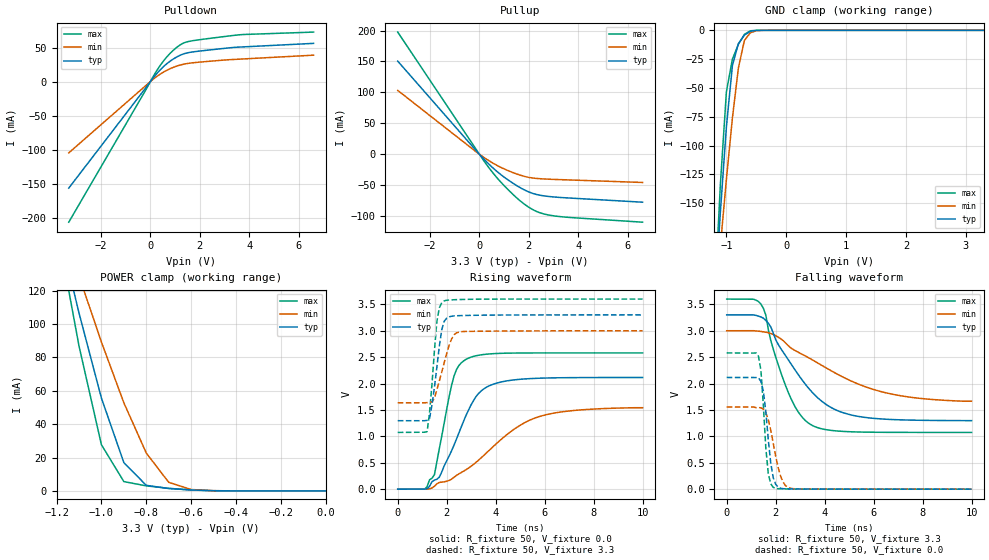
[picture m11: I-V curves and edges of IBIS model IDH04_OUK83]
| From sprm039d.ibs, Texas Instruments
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[Model]   IDH04_OUK83
Model_type   I/O
Vinh = 2.00
Vinl = 0.80
Enable   Active-Low
Polarity   Non-Inverting
| signals   A, GZ, Y
Vmeas = 1.5
|   typ   min   max
C_comp   2.356p   2.266p   2.394p
|   typ   min   max
[Temperature Range]   25   -40   125
|   typ   min   max
[Voltage Range]   3.30V   3.00V   3.60V
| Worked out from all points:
|   slope of the pulldown table from 0 to 0.495 V, typ, clamps not added: 23.8 ohm
|   slope of the pullup table from 0 to 0.495 V, typ, clamps not added: 24.4 ohm
|   GND clamp passes 1 mA (typ) near -0.61 V on its own axis
|   POWER clamp passes 1 mA (typ) near -0.65 V on its own axis
|   rising waveform, R_fixture 50, V_fixture 0.0: 20-80 % time 1.24ns typ, 2.52ns min, 658ps max; typ from 0 V to 2.12 V
|   falling waveform, R_fixture 50, V_fixture 3.3: 20-80 % time 1.85ns typ, 3.23ns min, 1.1ns max; typ from 3.3 V to 1.3 V
|   rising waveform, R_fixture 50, V_fixture 3.3: 20-80 % time 331ps typ, 486ps min, 260ps max; typ from 1.3 V to 3.3 V
|   falling waveform, R_fixture 50, V_fixture 0.0: 20-80 % time 285ps typ, 427ps min, 226ps max; typ from 2.12 V to 0 V
[Pulldown]
|   Voltage   I(typ)   I(min)   I(max)
-3.3V     -156.5mA   -104.8mA   -206.6mA
-200mV    -9.762mA   -6.342mA   -13.16mA
200mV     9.308mA    5.91mA     12.77mA
600mV     24.27mA    15.38mA    33.46mA
800mV     30.04mA    19mA       41.54mA
1.1V      36.8mA     23.15mA    51.22mA
1.3V      40.12mA    25.17mA    55.93mA
1.6V      42.95mA    27.12mA    59.33mA
3.5V      50.51mA    32.76mA    68.38mA
6.6V      56.15mA    38.81mA    72.73mA
[GND_clamp]
|   Voltage   I(typ)   I(min)   I(max)
-3.3V     -2.124A    -1.605A    -2.753A
-1.2V     -237.7mA   -246.3mA   -236.7mA
-1.1V     -157mA     -186.6mA   -132.9mA
-1V       -83.63mA   -129.2mA   -53.23mA
-900mV    -30.57mA   -76.17mA   -24.99mA
-800mV    -11.54mA   -32.67mA   -12.1mA
-700mV    -4.229mA   -8.865mA   -3.556mA
-600mV    -824.6uA   -2.094mA   -405.8uA
-500mV    -75.44uA   -369.7uA   -18.94uA
-400mV    -4.212uA   -45.39uA   -421.8nA
3.3V      310.9pA    1.955uA    0A
[Pullup]
|   Voltage   I(typ)   I(min)   I(max)
-3.3V     150.6mA    103.2mA    197.6mA
-200mV    9.015mA    6.05mA     12.03mA
300mV     -12.71mA   -8.337mA   -17.25mA
900mV     -34.06mA   -21.94mA   -46.59mA
1.4V      -48.08mA   -30.44mA   -66.63mA
1.8V      -57.38mA   -35.68mA   -80.27mA
2.3V      -65.13mA   -39.22mA   -92.49mA
2.9V      -68.83mA   -40.65mA   -99.12mA
3.7V      -71.1mA    -41.8mA    -102.6mA
6.6V      -77.74mA   -45.8mA    -110.1mA
[POWER_clamp]
|   Voltage   I(typ)   I(min)   I(max)
-3.3V     1.472A     1.113A     1.907A
-1.2V     162.8mA    170.3mA    159.8mA
-1.1V     106.7mA    128.9mA    86.98mA
-1V       55.67mA    89.28mA    27.7mA
-900mV    16.96mA    52.84mA    5.593mA
-800mV    3.336mA    22.68mA    3.033mA
-700mV    1.434mA    5.139mA    1.568mA
-600mV    594uA      840.3uA    550.9uA
-500mV    140.8uA    157.5uA    81.51uA
0V        1pA        1pA        1pA
[Ramp]
|   I(typ)   I(min)   I(max)
dV/dt_r   1.269/1.233n   0.927/2.522n   1.548/0.653n
dV/dt_f   1.201/1.853n   0.804/3.247n   1.515/1.097n
[Rising Waveform]
R_fixture = 50
V_fixture = 0.0
|  pu_on
|  TIME   V(typ)   V(min)   V(max)
0s        4nV        16nV       3nV
1.1ns     231.2uV    489.8uV    2.084mV
1.5ns     171.1mV    54.88mV    273.8mV
1.7ns     228.6mV    127.1mV    770.4mV
2.3ns     835.6mV    224.1mV    2.144V
2.8ns     1.408V     371.9mV    2.461V
3.2ns     1.755V     509.1mV    2.526V
3.7ns     1.949V     719.6mV    2.559V
5.7ns     2.1V       1.363V     2.58V
10ns      2.115V     1.542V     2.58V
[Falling Waveform]
R_fixture = 50
V_fixture = 3.3
V_fixture_min = 3.0
V_fixture_max = 3.6
|  pd_on
|  TIME   V(typ)   V(min)   V(max)
0s        3.3V       3V         3.6V
1.4ns     3.262V     2.986V     3.503V
1.6ns     3.196V     2.973V     3.295V
1.8ns     3.074V     2.949V     2.818V
2.5ns     2.462V     2.724V     1.85V
3ns       2.119V     2.574V     1.412V
3.5ns     1.831V     2.448V     1.206V
4.4ns     1.514V     2.208V     1.106V
5.4ns     1.376V     1.986V     1.083V
10ns      1.298V     1.665V     1.075V
[Rising Waveform]
R_fixture = 50
V_fixture = 3.3
V_fixture_min = 3.0
V_fixture_max = 3.6
|  pd_off
|  TIME   V(typ)   V(min)   V(max)
0s        1.297V     1.636V     1.075V
1.2ns     1.303V     1.639V     1.09V
1.3ns     1.339V     1.645V     1.447V
1.5ns     1.932V     1.726V     2.627V
1.6ns     2.315V     1.883V     3.182V
1.8ns     3.023V     2.221V     3.533V
1.9ns     3.18V      2.398V     3.566V
2.2ns     3.275V     2.844V     3.585V
2.6ns     3.287V     2.983V     3.592V
10ns      3.3V       3V         3.6V
[Falling Waveform]
R_fixture = 50
V_fixture = 0.0
|  pu_off
|  TIME   V(typ)   V(min)   V(max)
0s        2.115V     1.555V     2.58V
1.3ns     2.108V     1.544V     2.516V
1.4ns     2.038V     1.541V     2.243V
1.5ns     1.853V     1.516V     1.567V
1.6ns     1.457V     1.446V     768.9mV
1.7ns     935mV      1.313V     289.4mV
1.9ns     221mV      872.5mV    36.25mV
2.2ns     17.19mV    250.2mV    7.117mV
2.6ns     5.715mV    16.9mV     3.594mV
10ns      3.96uV     94.7uV     12.14uV
